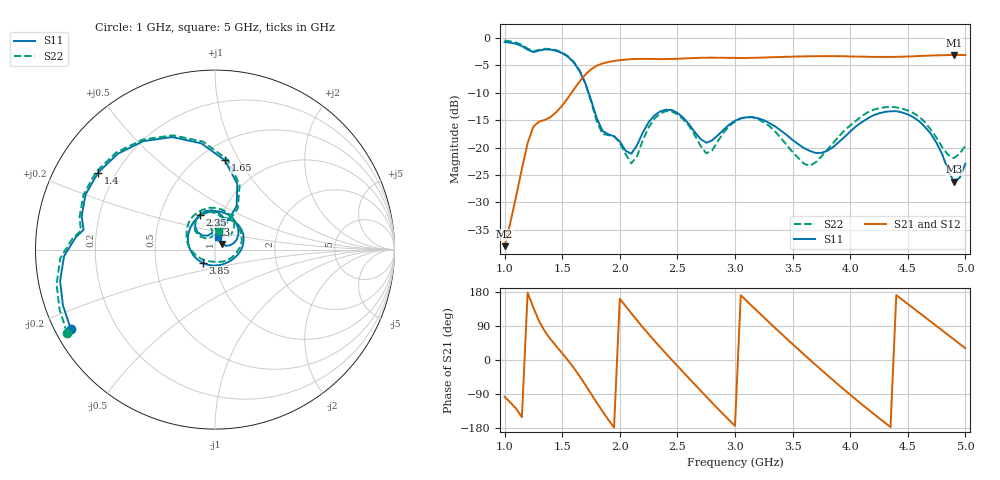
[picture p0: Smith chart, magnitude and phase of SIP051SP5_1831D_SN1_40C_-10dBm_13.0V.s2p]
# GHz  S  dB  R  50
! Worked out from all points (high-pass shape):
!   81 points, 1 GHz to 5 GHz, reference 50 ohm
!   highest |S21| = -3.13 dB at 4.9 GHz (marker M1); lowest = -38.0 dB at 1 GHz (marker M2)
!   |S21| within 3 dB of the highest: 1.73 GHz to end of sweep
!   lowest |S11| = -26.2 dB at 4.9 GHz (marker M3), VSWR 1.10, Z = 53.9 + j3.3 ohm
!   |S11| at or under -10 dB: 1.729 GHz to end of sweep
!   |S22| runs from -23.3 to -0.5 dB; largest |S21 - S12| = 0.002
!   S11 on the Smith chart (normalised r, x): 1 GHz: 0.05, -0.26; 1.4 GHz: 0.13, +0.30; 1.65 GHz: 0.66, +0.87; 2.35 GHz: 0.78, +0.32; 3.85 GHz: 0.87, -0.13; 5 GHz: 1.03, +0.14
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1  -0.76 -151.3  -37.98 -97.1  -37.93 -98.5  -0.48 -150.6
1.25  -2.61 171.4  -16.18 137.8  -16.20 137.6  -2.45 172.0
1.4  -2.16 146.6  -14.43 54.4  -14.42 54.4  -2.03 146.7
1.65  -6.02 83.6  -8.00 -42.3  -7.98 -42.2  -5.91 82.1
1.7  -8.25 71.3  -6.72 -65.3  -6.73 -65.2  -8.25 69.2
1.8  -14.65 65.5  -5.09 -112.7  -5.09 -112.7  -15.24 63.8
2  -18.91 92.1  -4.08 161.7  -4.08 161.8  -19.13 88.6
2.15  -19.57 131.4  -3.85 104.5  -3.85 104.4  -21.58 131.4
2.35  -13.42 113.7  -3.88 34.0  -3.88 33.9  -13.82 118.9
2.5  -13.69 84.7  -3.82 -15.6  -3.82 -15.6  -13.94 86.9
2.7  -18.42 71.4  -3.64 -80.4  -3.64 -80.4  -19.67 69.2
3  -15.12 73.5  -3.66 -173.9  -3.65 -174.0  -15.24 84.5
3.2  -14.67 36.8  -3.63 127.1  -3.63 127.1  -14.82 41.6
3.35  -16.15 7.2  -3.52 84.0  -3.53 84.0  -17.11 5.3
3.55  -19.39 -35.3  -3.40 28.0  -3.40 28.0  -21.92 -56.2
3.7  -20.98 -77.9  -3.35 -13.0  -3.35 -12.9  -22.68 -117.8
3.85  -19.95 -131.9  -3.34 -52.8  -3.35 -52.8  -19.22 -162.4
4.05  -16.14 165.1  -3.42 -104.2  -3.42 -104.2  -15.13 154.9
4.35  -13.39 92.0  -3.49 -177.1  -3.50 -177.1  -12.57 98.0
4.65  -16.27 32.2  -3.28 112.8  -3.28 112.9  -15.42 50.6
4.9  -26.21 38.7  -3.13 54.3  -3.13 54.3  -21.92 61.8
5  -22.93 74.3  -3.14 31.1  -3.15 31.1  -19.67 77.6
